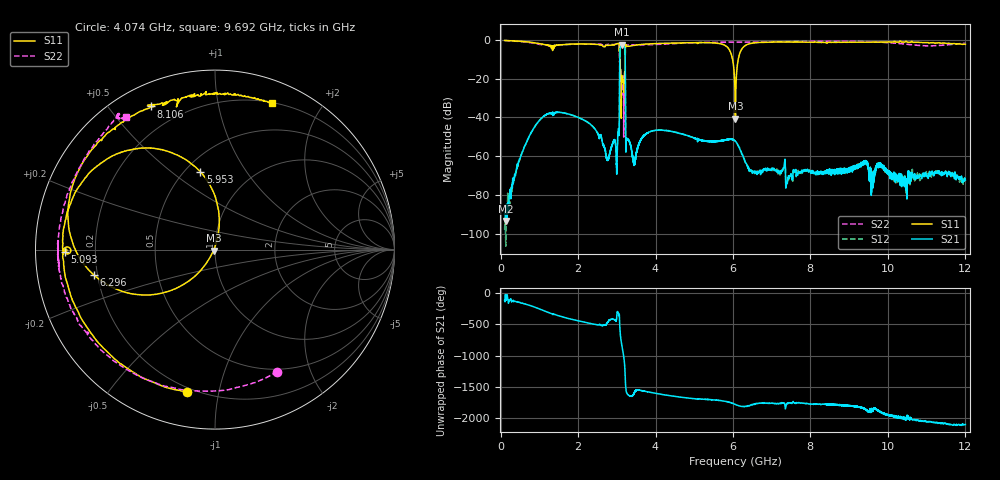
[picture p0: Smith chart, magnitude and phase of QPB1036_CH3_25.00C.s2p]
! TDS: K:\Engsetup\Winsaw\QPB1036_ALL
! Channel 1
! Ports=1 2
! seg 1=100.000000 1100.000000 101
! seg 2=1101.000000 1501.000000 401
! seg 3=1502.000000 2502.000000 101
! seg 4=2503.000000 3803.000000 1301
! seg 5=3804.000000 5004.000000 121
! seg 6=5005.000000 6005.000000 1001
! seg 7=6006.000000 8406.000000 241
! seg 8=8407.000000 10607.000000 2201
! seg 9=10608.000000 12008.000000 141
! Points=5609
! FailCode=0
! Topology=ALL_SE(12)
!VNA Cal loaded =QPB1036_ALL_25C
!PS1(V)= 5.000
!PS(mA)= 0.500
!PS2(V)= 0.630
!PS(mA)= -0.100
!PS3(V)= 1.170
!PS(mA)= 0.100
!PS4(V)= 1.170
!PS(mA)= -0.100
!Temp (C)= 25.00
# MHz S DB R 50
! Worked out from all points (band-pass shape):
!   5609 points, 100 MHz to 12.01 GHz, reference 50 ohm
!   highest |S21| = -2.44 dB at 3.13 GHz (marker M1); lowest = -93.5 dB at 130 MHz (marker M2)
!   |S21| within 3 dB of the highest: 3.083 GHz to 3.213 GHz (130.2 MHz wide, 4.14 % of centre)
!   lowest |S11| = -40.7 dB at 6.066 GHz (marker M3), VSWR 1.02, Z = 49.2 - j0.504 ohm
!   |S11| at or under -10 dB: 3.083 GHz to 3.216 GHz (132.9 MHz wide, 4.22 % of centre); 5.991 GHz to 6.138 GHz (147.6 MHz wide, 2.43 % of centre)
!   |S22| runs from -50.1 to -0.3 dB; largest |S21 - S12| = 0.0053
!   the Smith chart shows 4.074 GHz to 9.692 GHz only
!   S11 on the Smith chart (normalised r, x): 4.074 GHz: 0.18, -0.81; 5.093 GHz: 0.09, -0.01; 5.953 GHz: 0.59, +0.64; 6.296 GHz: 0.19, -0.10; 8.106 GHz: 0.10, +0.64; 9.692 GHz: 0.20, +1.44
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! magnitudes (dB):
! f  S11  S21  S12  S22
! 100 MHz  -0.3  -90.1  -98.0  -0.3
! 130 MHz  -0.3  -93.5  -106.4  -0.3
! 1.127 GHz  -2.5  -39.1  -39.2  -2.6
! 2.092 GHz  -2.1  -40.8  -40.8  -2.2
! 2.992 GHz  -2.1  -64.6  -64.4  -2.0
! 3.037 GHz  -1.8  -46.4  -46.3  -2.0
! 3.095 GHz  -15.1  -3.3  -3.2  -17.8
! 3.13 GHz  -18.6  -2.4  -2.4  -27.1
! 3.194 GHz  -20.1  -3.4  -3.3  -18.4
! 3.255 GHz  -3.1  -50.8  -51.0  -2.7
! 3.44 GHz  -2.8  -64.1  -64.1  -2.5
! 4.074 GHz  -1.9  -46.6  -46.5  -2.3
! 5.093 GHz  -1.5  -51.6  -51.5  -1.4
! 5.953 GHz  -7.1  -51.1  -51.1  -1.2
! 6.056 GHz  -28.3  -52.1  -52.1  -1.2
! 6.066 GHz  -40.7  -52.4  -52.3  -1.2
! 6.296 GHz  -3.2  -61.9  -61.4  -1.2
! 8.046 GHz  -1.2  -67.3  -67.8  -0.7
! 8.106 GHz  -1.2  -68.8  -68.4  -0.7
! 9.692 GHz  -1.1  -67.2  -65.8  -1.0
! 10.02 GHz  -0.9  -68.2  -69.5  -1.5
! 12.01 GHz  -2.3  -72.4  -71.8  -1.7
